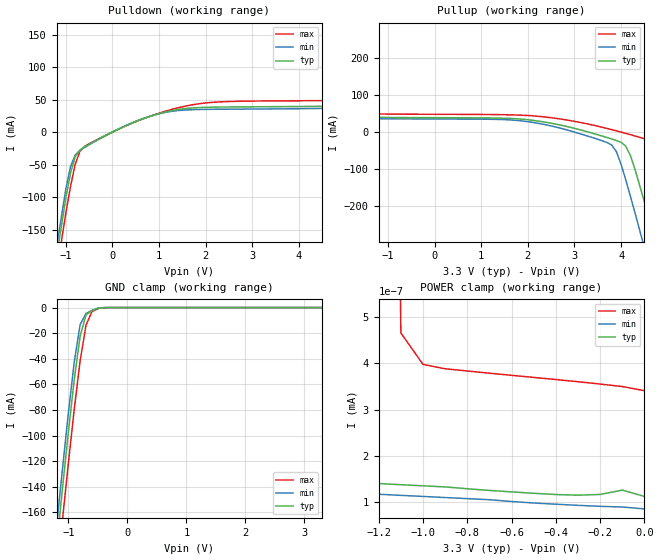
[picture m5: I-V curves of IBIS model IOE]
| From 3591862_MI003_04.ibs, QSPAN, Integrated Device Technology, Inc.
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|   Model IOE
[Model]   IOE
Model_type   I/O
Polarity   Non-Inverting
Vinl =   0.8000V
Vinh =   2.0000V
C_comp   5.0000pF   5.0000pF   5.0000pF
[Temperature Range]   27.0000   0.000   70.0000
[Voltage Range]   3.3000V   3.0000V   4.0000V
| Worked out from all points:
|   slope of the pulldown table from 0 to 0.495 V, typ, clamps not added: 30.8 ohm
|   slope of the pullup table from 0 to 0.495 V, typ, clamps not added: 2.18 kohm
|   GND clamp passes 1 mA (typ) near -0.52 V on its own axis
|   POWER clamp passes 1 mA (typ) near -2.42 V on its own axis
[Pulldown]
| voltage   I(typ)   I(min)   I(max)
-3.3V     -1.194A    -1.18A     -1.216A
-1.5V     -327.8mA   -312.7mA   -352mA
-1V       -101.3mA   -87.47mA   -124.6mA
-900mV    -63.38mA   -53.14mA   -83.81mA
-800mV    -37.91mA   -35.22mA   -49.72mA
-700mV    -27.61mA   -28.33mA   -29.79mA
-600mV    -22.79mA   -23.79mA   -22.13mA
800mV     23.97mA    24.19mA    24.19mA
2.1V      38.27mA    35.04mA    45.53mA
5.7V      43.18mA    40.4mA     52.16mA
5.9V      59.6mA     52.73mA    74.14mA
6.6V      176.3mA    169.7mA    189.7mA
[Pullup]
| voltage   I(typ)   I(min)   I(max)
-3.3V     176.3mA    117.1mA    314.7mA
-2.5V     47.69mA    39.24mA    172.5mA
-1.7V     40.43mA    36.75mA    52.16mA
1.8V      35.65mA    31.16mA    46.02mA
3.7V      -14.76mA   -28.33mA   9.93mA
3.9V      -22.79mA   -53.14mA   3.442mA
4.1V      -37.91mA   -129.2mA   -3.465mA
4.5V      -188.7mA   -312.7mA   -17.89mA
4.7V      -280.9mA   -407.5mA   -29.79mA
5.3V      -565.7mA   -695.6mA   -258.8mA
5.5V      -661.9mA   -792.3mA   -352mA
6.6V      -1.194A    -1.326A    -878mA
[GND_clamp]
| voltage   I(typ)   I(min)   I(max)
-3.3V     -1.194A    -1.18A     -1.216A
-1.2V     -186.9mA   -171.6mA   -211.6mA
-1.1V     -141.6mA   -126.3mA   -166.2mA
-1V       -97.58mA   -82.55mA   -121.9mA
-900mV    -56.31mA   -42.52mA   -79.6mA
-800mV    -22.23mA   -13.2mA    -41.49mA
-700mV    -5.772mA   -4.585mA   -13.66mA
-600mV    -2.251mA   -2.179mA   -3.176mA
-500mV    -602.5uA   -505.7uA   -793.8uA
-300mV    -1.593uA   -434.4nA   -7.283uA
3.3V      109.9pA    95.94pA    356.2pA
[POWER_clamp]
| voltage   I(typ)   I(min)   I(max)
-3.3V     126.9mA    72.49mA    251.8mA
-2.4V     364.9uA    8.299nA    101.6mA
-2.3V     32.02uA    292.1pA    85.28mA
-2.2V     1.772uA    171.7pA    69.15mA
-2.1V     73.02nA    144.1pA    53.29mA
-2V       3.241nA    137.8pA    37.83mA
-1.9V     237.4pA    135.1pA    23.2mA
-1.8V     171.9pA    132.5pA    10.25mA
-1.7V     155pA      130pA      1.958mA
-1.2V     140.7pA    117.6pA    4.879nA
-1V       135.8pA    112.9pA    397.7pA
0V        113pA      86.05pA    341pA
[Ramp]
|variable
dV/dt_r   0/0   0/0   0/0
dV/dt_f   1.0776/0.1236n   0.9864/0.1153n   1.2888/0.1264n
R_load = 50.0000
| End [Model] IOE
